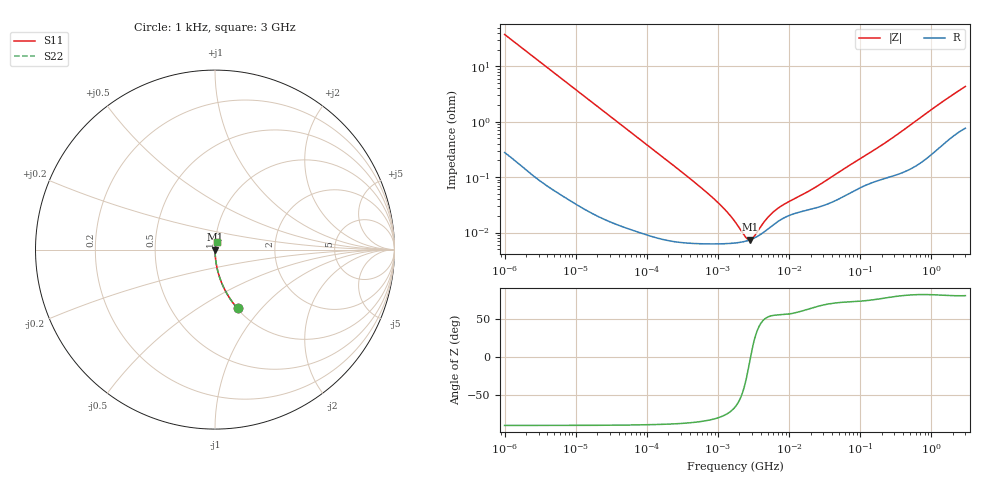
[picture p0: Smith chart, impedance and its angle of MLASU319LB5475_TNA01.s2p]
! MLASU319LB5475_TNA01  S-PARAMETER MODEL  ( Standard Model )
! Model Generated by TAIYO YUDEN Corporation (http://www.ty-top.com)
! Version 1.0
! TAIYO YUDEN Control No. 220601
! Copyright(c) 2010 TAIYO YUDEN CO.,LTD. All Rights Reserved.
! Product Description (link to TY-COMPAS)
! https://ds.yuden.co.jp/TYCOMPAS/or/detail?pn=MLASU319LB5475KTNA01&u=M
! Products Name : Multilayer Ceramic Capacitors
! Characteristics :
!  Capacitance : 4.7 [uF] , Rated Voltage : 50 [V] , TCC : X5R
!  Case Size : 3.2 x 1.6 / 0.126 x 0.063 [mm/inch] , Thickness : 0.85 / 0.033 [mm/inch]
!  (Conditions: Temperature = 25 [degC] , DC Bias Voltage = 0 [V])
! External Node Assignments :
!  1  o---| |---o  2
! GND o---------o GND
! Frequency Range : 1kHz  -  3GHz  [ 401 STEP ]
# MHZ S RI R 50
! Freq[MHz].  S11 Real  S11 Imag  S21 Real  S21 Imag  S12 Real  S12 Imag  S22 Real  S22 Imag
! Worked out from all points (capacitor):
!   401 points, 1 kHz to 3 GHz, reference 50 ohm
!   read as one part in series: C = 4.23 uF near 1.077 kHz
!   lowest |Z| = 7.4 mohm at 2.812 MHz (marker M1)
!   series resonance near 2.872 MHz, so ESL is about 730 pH
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0.001  0.1256 -0.3277  0.8744 0.3277  0.8744 0.3277  0.1256 -0.3277
0.001685  0.049 -0.2123  0.951 0.2123  0.951 0.2123  0.049 -0.2123
0.00306  0.0158 -0.1214  0.9842 0.1214  0.9842 0.1214  0.0158 -0.1214
0.005768  0.00479 -0.0653  0.9952 0.0653  0.9952 0.0653  0.00479 -0.0653
0.01216  0.00125 -0.0312  0.9987 0.0312  0.9987 0.0312  0.00125 -0.0312
0.147855  8.47e-05 -0.0026  0.9999 0.0026  0.9999 0.0026  8.47e-05 -0.0026
0.419985  6.45e-05 -0.000901  0.9999 0.000901  0.9999 0.000901  6.45e-05 -0.000901
0.791611  6.24e-05 -0.000452  0.9999 0.000452  0.9999 0.000452  6.24e-05 -0.000452
1.238299  6.29e-05 -0.000255  0.9999 0.000255  0.9999 0.000255  6.29e-05 -0.000255
1.732051  6.47e-05 -0.000143  0.9999 0.000143  0.9999 0.000143  6.47e-05 -0.000143
2.087011  6.68e-05 -8.81e-05  0.9999 8.81e-05  0.9999 8.81e-05  6.68e-05 -8.81e-05
2.24859  6.8e-05 -6.71e-05  0.9999 6.71e-05  0.9999 6.71e-05  6.8e-05 -6.71e-05
2.812335  7.37e-05 -5.65e-06  0.9999 5.65e-06  0.9999 5.65e-06  7.37e-05 -5.65e-06
3.264662  8e-05 3.46e-05  0.9999 -3.46e-05  0.9999 -3.46e-05  8e-05 3.46e-05
3.517417  8.41e-05 5.47e-05  0.9999 -5.47e-05  0.9999 -5.47e-05  8.41e-05 5.47e-05
5.106836  0.000117 0.000152  0.9999 -0.000152  0.9999 -0.000152  0.000117 0.000152
5.928204  0.000136 0.000188  0.9999 -0.000188  0.9999 -0.000188  0.000136 0.000188
7.143107  0.000162 0.00023  0.9998 -0.00023  0.9998 -0.00023  0.000162 0.00023
21.06097  0.000267 0.000543  0.9997 -0.000543  0.9997 -0.000543  0.000267 0.000543
256.0921  0.00102 0.00456  0.999 -0.00456  0.999 -0.00456  0.00102 0.00456
1371.11  0.00408 0.0217  0.9959 -0.0217  0.9959 -0.0217  0.00408 0.0217
3000  0.00935 0.042  0.9906 -0.042  0.9906 -0.042  0.00935 0.042
